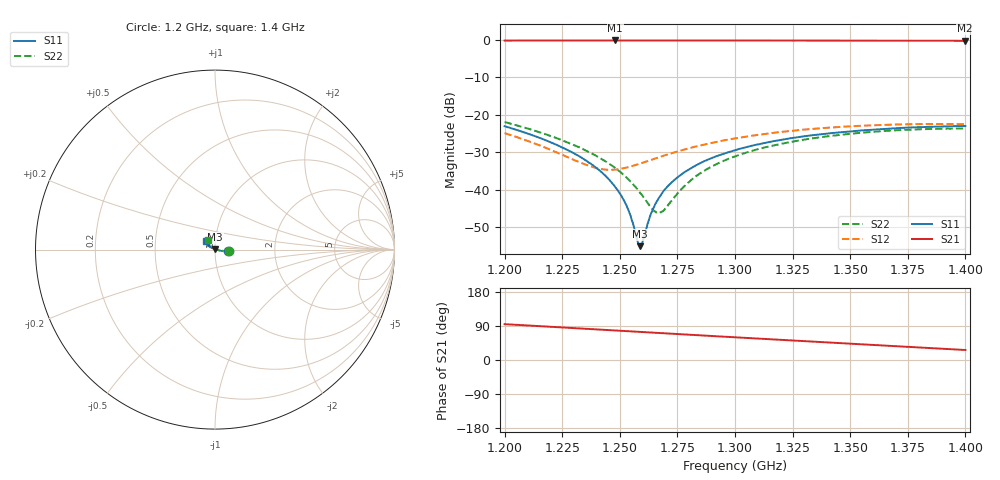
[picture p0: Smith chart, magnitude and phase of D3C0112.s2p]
! 11/4/2020 8:25:18 AM
! C:\USERS\DITOM\DESKTOP\SINGLE JUNCTION ISOLATOR DATA\1.2-1.4 GHZ (D3I0112).S2P
! CHANNEL.1
! TR.MEASUREMENT
! CORRECTED.DATA
# GHZ S RI R 50.0
! FREQ.GHZ  S11RE  S11IM  S21RE  S21IM  S12RE  S12IM  S22RE  S22IM
!; PortSelection: Port_12
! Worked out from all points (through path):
!   601 points, 1.2 GHz to 1.4 GHz, reference 50 ohm
!   highest |S21| = -0.11 dB at 1.248 GHz (marker M1); lowest = -0.2 dB at 1.4 GHz (marker M2)
!   lowest |S11| = -55.1 dB at 1.259 GHz (marker M3), VSWR 1.00, Z = 50.1 + j0.159 ohm
!   |S11| at or under -10 dB: start of sweep to end of sweep
!   |S22| runs from -46.2 to -21.9 dB; largest |S21 - S12| = 0.97
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1.2  0.0698 -0.0103  -0.0785 0.9801  0.0488 0.0295  0.0795 -0.0102
1.219  0.0435 -0.00823  0.037 0.9852  0.029 0.0198  0.0529 -0.00816
1.233667  0.0259 -0.00537  0.1265 0.9783  0.0145 0.0173  0.0348 -0.00522
1.241667  0.0172 -0.00327  0.1745 0.9713  0.00709 0.0176  0.026 -0.0033
1.248  0.0107 -0.00161  0.2118 0.9643  0.00169 0.0185  0.0195 -0.00155
1.253333  0.00567 -0.000119  0.2423 0.9568  -0.00249 0.0198  0.0142 8.08e-05
1.255  0.00408 0.000443  0.2519 0.9543  -0.00376 0.0202  0.0126 0.000537
1.257667  0.00166 0.00132  0.267 0.9503  -0.00579 0.021  0.01 0.00143
1.258667  0.000754 0.00159  0.2727 0.9485  -0.00651 0.0213  0.00905 0.00181
1.259667  -0.00018 0.00189  0.2784 0.9469  -0.00716 0.0216  0.00817 0.00214
1.263333  -0.00351 0.00303  0.2991 0.9403  -0.00964 0.0229  0.00488 0.00336
1.266667  -0.0063 0.00404  0.3175 0.934  -0.0117 0.0243  0.00198 0.00448
1.268667  -0.008 0.00477  0.3287 0.9298  -0.0128 0.0251  0.00028 0.00513
1.271333  -0.0101 0.00561  0.3434 0.9244  -0.0143 0.0263  -0.00192 0.00619
1.279  -0.0158 0.00839  0.3848 0.9076  -0.0181 0.0301  -0.00806 0.00884
1.288333  -0.0225 0.0116  0.4338 0.8846  -0.0215 0.0351  -0.0146 0.0125
1.3  -0.0298 0.0159  0.4935 0.8523  -0.0242 0.0419  -0.022 0.0172
1.313333  -0.0368 0.0211  0.5586 0.8106  -0.0248 0.0499  -0.029 0.0228
1.333667  -0.0451 0.0288  0.651 0.7377  -0.0213 0.0614  -0.0368 0.0317
1.366667  -0.0515 0.0404  0.7778 0.5967  -0.00544 0.0736  -0.0421 0.0446
1.399667  -0.0514 0.0489  0.8748 0.4363  0.0159 0.0733  -0.0396 0.0526
1.4  -0.0513 0.049  0.8757 0.4347  0.0161 0.0733  -0.0396 0.0525
